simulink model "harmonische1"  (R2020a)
settings: Solver=ode45  StartTime=-8  StopTime=8  MaxStep=0.01  RelTol=1e-3  EnableMultiTasking=on

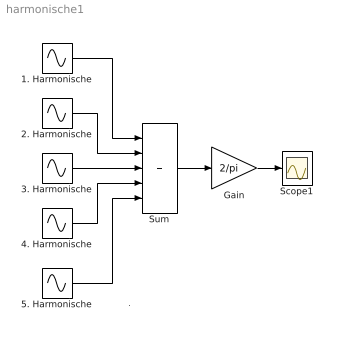
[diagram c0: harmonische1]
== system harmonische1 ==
  note: .
  1. Harmonische : Sin  SampleTime=0
  2. Harmonische : Sin  Amplitude=1/2  Frequency=2  SampleTime=0
  3. Harmonische : Sin  Amplitude=1/3  Frequency=3  SampleTime=0
  4. Harmonische : Sin  Amplitude=1/4  Frequency=4  SampleTime=0
  5. Harmonische : Sin  Amplitude=1/5  Frequency=5  SampleTime=0
  Gain : Gain  Gain=2/pi  SaturateOnIntegerOverflow=on
  Scope1 : Scope
  Sum : Sum  Inputs=5  SaturateOnIntegerOverflow=on
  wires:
  Gain/1 -> Scope1/1
  Sum/1 -> Gain/1
  3. Harmonische/1 -> Sum/3
  2. Harmonische/1 -> Sum/2
  1. Harmonische/1 -> Sum/1
  4. Harmonische/1 -> Sum/4
  5. Harmonische/1 -> Sum/5
